PROGRAM P_Prog4
VAR

	fbKL6401 					: FB_LON_KL6401;

	fbREAD_094		: FB_READ_094_SNVT_preset;
	fbSEND_094		: FB_SEND_094_SNVT_preset;

	fbREAD_095		: FB_READ_095_SNVT_switch;
	fbSEND_095		: FB_SEND_095_SNVT_switch;

	fbREAD_096		: FB_READ_096_SNVT_trans_table;
	fbSEND_096		: FB_SEND_096_SNVT_trans_table;

	fbREAD_097		: FB_READ_097_SNVT_override;
	fbSEND_097		: FB_SEND_097_SNVT_override;

	fbREAD_098		: FB_READ_098_SNVT_pwr_fact;
	fbSEND_098		: FB_SEND_098_SNVT_pwr_fact;

	fbREAD_099		: FB_READ_099_SNVT_pwr_fact_f;
	fbSEND_099		: FB_SEND_099_SNVT_pwr_fact_f;

	fbREAD_100		: FB_READ_100_SNVT_density;
	fbSEND_100		: FB_SEND_100_SNVT_density;

	fbREAD_101		: FB_READ_101_SNVT_density_f;
	fbSEND_101		: FB_SEND_101_SNVT_density_f;

	fbREAD_102		: FB_READ_102_SNVT_rpm;
	fbSEND_102		: FB_SEND_102_SNVT_rpm;

	fbREAD_103		: FB_READ_103_SNVT_hvac_emerg;
	fbSEND_103		: FB_SEND_103_SNVT_hvac_emerg;

	fbREAD_104		: FB_READ_104_SNVT_angle_deg;
	fbSEND_104		: FB_SEND_104_SNVT_angle_deg;

	fbREAD_105		: FB_READ_105_SNVT_temp_p;
	fbSEND_105		: FB_SEND_105_SNVT_temp_p;

	fbREAD_106		: FB_READ_106_SNVT_temp_setpt;
	fbSEND_106		: FB_SEND_106_SNVT_temp_setpt;

	fbREAD_107		: FB_READ_107_SNVT_time_sec;
	fbSEND_107		: FB_SEND_107_SNVT_time_sec;

	fbREAD_108		: FB_READ_108_SNVT_hvac_mode;
	fbSEND_108		: FB_SEND_108_SNVT_hvac_mode;

	fbREAD_109		: FB_READ_109_SNVT_occupancy;
	fbSEND_109		: FB_SEND_109_SNVT_occupancy;

	fbREAD_110		: FB_READ_110_SNVT_area;
	fbSEND_110		: FB_SEND_110_SNVT_area;

	fbREAD_111		: FB_READ_111_SNVT_hvac_overid;
	fbSEND_111		: FB_SEND_111_SNVT_hvac_overid;

	fbREAD_112		: FB_READ_112_SNVT_hvac_status;
	fbSEND_112		: FB_SEND_112_SNVT_hvac_status;

	fbREAD_113		: FB_READ_113_SNVT_press_p;
	fbSEND_113		: FB_SEND_113_SNVT_press_p;

	fbREAD_114		: FB_READ_114_SNVT_address;
	fbSEND_114		: FB_SEND_114_SNVT_address;

	fbREAD_115		: FB_READ_115_SNVT_scene;
	fbSEND_115		: FB_SEND_115_SNVT_scene;

	fbREAD_116		: FB_READ_116_SNVT_scene_cfg;
	fbSEND_116		: FB_SEND_116_SNVT_scene_cfg;

	fbREAD_117		: FB_READ_117_SNVT_setting;
	fbSEND_117		: FB_SEND_117_SNVT_setting;

	fbREAD_118		: FB_READ_118_SNVT_evap_state;
	fbSEND_118		: FB_SEND_118_SNVT_evap_state;

	fbREAD_119		: FB_READ_119_SNVT_therm_mode;
	fbSEND_119		: FB_SEND_119_SNVT_therm_mode;

	fbREAD_120		: FB_READ_120_SNVT_defr_mode;
	fbSEND_120		: FB_SEND_120_SNVT_defr_mode;

	fbREAD_121		: FB_READ_121_SNVT_defr_term;
	fbSEND_121		: FB_SEND_121_SNVT_defr_term;

	fbREAD_122		: FB_READ_122_SNVT_defr_state;
	fbSEND_122		: FB_SEND_122_SNVT_defr_state;

	fbREAD_123		: FB_READ_123_SNVT_time_min;
	fbSEND_123		: FB_SEND_123_SNVT_time_min;

	fbREAD_124		: FB_READ_124_SNVT_time_hour;
	fbSEND_124		: FB_SEND_124_SNVT_time_hour;

END_VAR

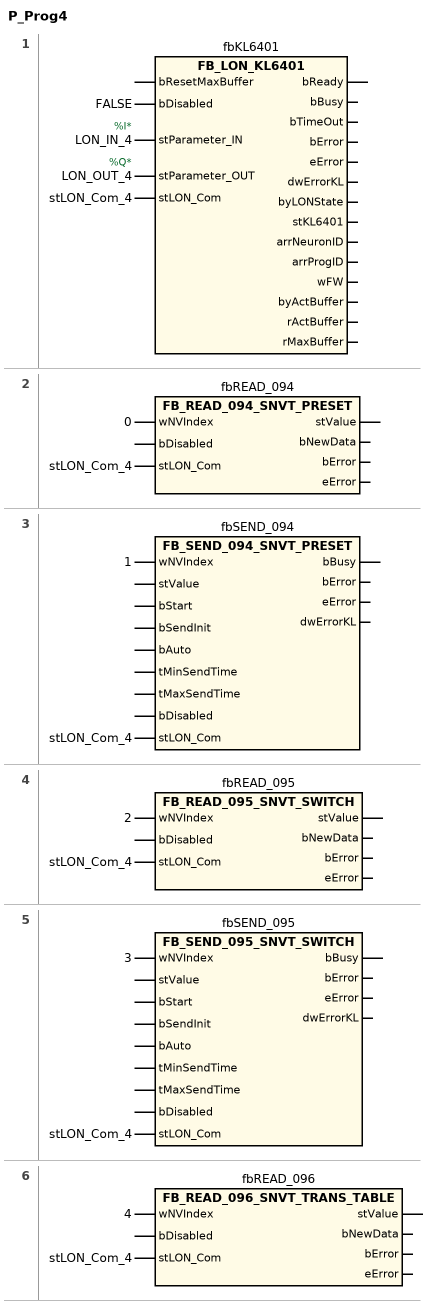
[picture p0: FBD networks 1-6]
// NETWORK 1
//   LON_IN_4: AT %I*
//   LON_OUT_4: AT %Q*
fbKL6401(
    bDisabled := FALSE,
    stParameter_IN := LON_IN_4,
    stParameter_OUT := LON_OUT_4,
    stLON_Com := stLON_Com_4); // FB_LON_KL6401

// NETWORK 2
fbREAD_094(wNVIndex := 0, stLON_Com := stLON_Com_4); // FB_READ_094_SNVT_PRESET

// NETWORK 3
fbSEND_094(wNVIndex := 1, stLON_Com := stLON_Com_4); // FB_SEND_094_SNVT_PRESET

// NETWORK 4
fbREAD_095(wNVIndex := 2, stLON_Com := stLON_Com_4); // FB_READ_095_SNVT_SWITCH

// NETWORK 5
fbSEND_095(wNVIndex := 3, stLON_Com := stLON_Com_4); // FB_SEND_095_SNVT_SWITCH

// NETWORK 6
fbREAD_096(wNVIndex := 4, stLON_Com := stLON_Com_4); // FB_READ_096_SNVT_TRANS_TABLE

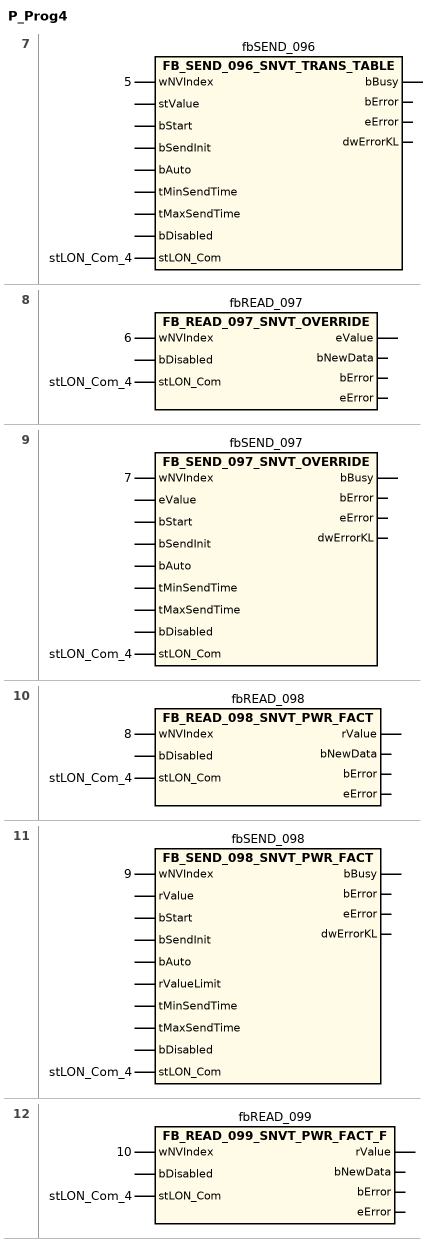
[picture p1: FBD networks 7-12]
// NETWORK 7
fbSEND_096(wNVIndex := 5, stLON_Com := stLON_Com_4); // FB_SEND_096_SNVT_TRANS_TABLE

// NETWORK 8
fbREAD_097(wNVIndex := 6, stLON_Com := stLON_Com_4); // FB_READ_097_SNVT_OVERRIDE

// NETWORK 9
fbSEND_097(wNVIndex := 7, stLON_Com := stLON_Com_4); // FB_SEND_097_SNVT_OVERRIDE

// NETWORK 10
fbREAD_098(wNVIndex := 8, stLON_Com := stLON_Com_4); // FB_READ_098_SNVT_PWR_FACT

// NETWORK 11
fbSEND_098(wNVIndex := 9, stLON_Com := stLON_Com_4); // FB_SEND_098_SNVT_PWR_FACT

// NETWORK 12
fbREAD_099(wNVIndex := 10, stLON_Com := stLON_Com_4); // FB_READ_099_SNVT_PWR_FACT_F

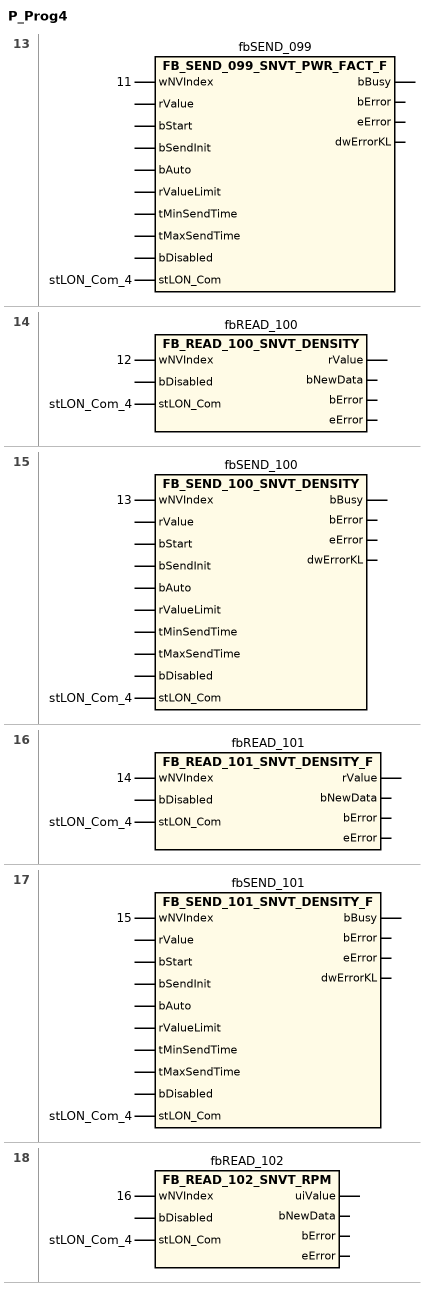
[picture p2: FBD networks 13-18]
// NETWORK 13
fbSEND_099(wNVIndex := 11, stLON_Com := stLON_Com_4); // FB_SEND_099_SNVT_PWR_FACT_F

// NETWORK 14
fbREAD_100(wNVIndex := 12, stLON_Com := stLON_Com_4); // FB_READ_100_SNVT_DENSITY

// NETWORK 15
fbSEND_100(wNVIndex := 13, stLON_Com := stLON_Com_4); // FB_SEND_100_SNVT_DENSITY

// NETWORK 16
fbREAD_101(wNVIndex := 14, stLON_Com := stLON_Com_4); // FB_READ_101_SNVT_DENSITY_F

// NETWORK 17
fbSEND_101(wNVIndex := 15, stLON_Com := stLON_Com_4); // FB_SEND_101_SNVT_DENSITY_F

// NETWORK 18
fbREAD_102(wNVIndex := 16, stLON_Com := stLON_Com_4); // FB_READ_102_SNVT_RPM

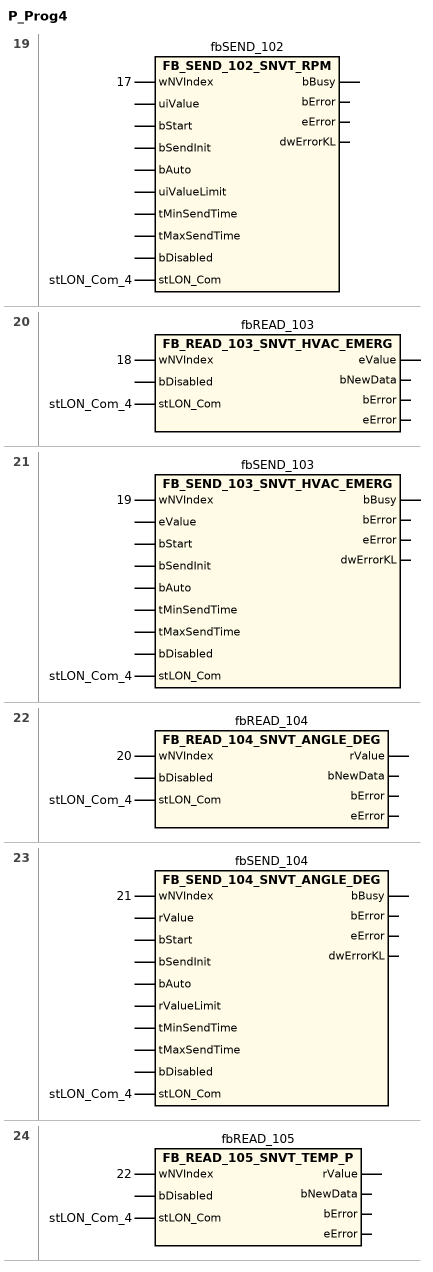
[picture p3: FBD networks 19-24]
// NETWORK 19
fbSEND_102(wNVIndex := 17, stLON_Com := stLON_Com_4); // FB_SEND_102_SNVT_RPM

// NETWORK 20
fbREAD_103(wNVIndex := 18, stLON_Com := stLON_Com_4); // FB_READ_103_SNVT_HVAC_EMERG

// NETWORK 21
fbSEND_103(wNVIndex := 19, stLON_Com := stLON_Com_4); // FB_SEND_103_SNVT_HVAC_EMERG

// NETWORK 22
fbREAD_104(wNVIndex := 20, stLON_Com := stLON_Com_4); // FB_READ_104_SNVT_ANGLE_DEG

// NETWORK 23
fbSEND_104(wNVIndex := 21, stLON_Com := stLON_Com_4); // FB_SEND_104_SNVT_ANGLE_DEG

// NETWORK 24
fbREAD_105(wNVIndex := 22, stLON_Com := stLON_Com_4); // FB_READ_105_SNVT_TEMP_P

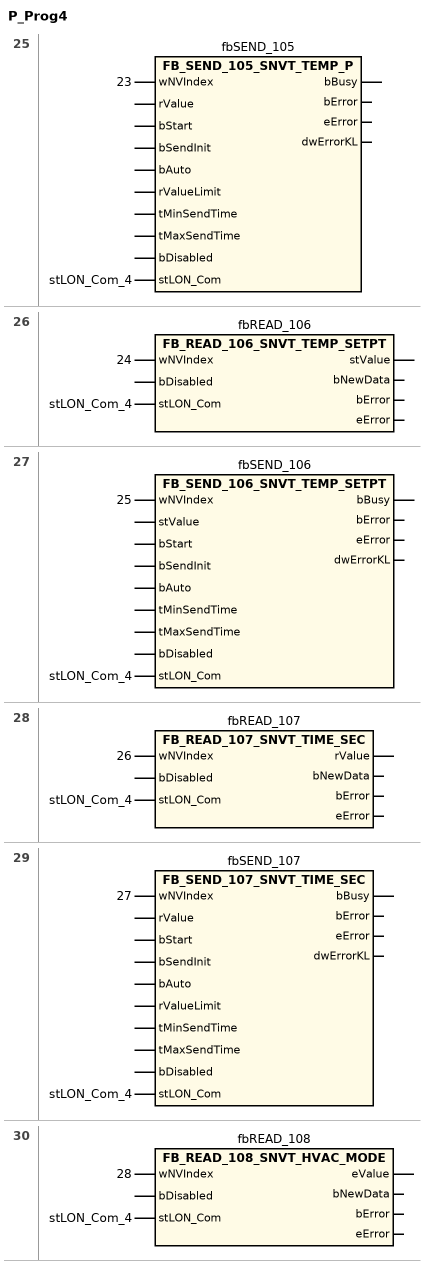
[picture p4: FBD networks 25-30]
// NETWORK 25
fbSEND_105(wNVIndex := 23, stLON_Com := stLON_Com_4); // FB_SEND_105_SNVT_TEMP_P

// NETWORK 26
fbREAD_106(wNVIndex := 24, stLON_Com := stLON_Com_4); // FB_READ_106_SNVT_TEMP_SETPT

// NETWORK 27
fbSEND_106(wNVIndex := 25, stLON_Com := stLON_Com_4); // FB_SEND_106_SNVT_TEMP_SETPT

// NETWORK 28
fbREAD_107(wNVIndex := 26, stLON_Com := stLON_Com_4); // FB_READ_107_SNVT_TIME_SEC

// NETWORK 29
fbSEND_107(wNVIndex := 27, stLON_Com := stLON_Com_4); // FB_SEND_107_SNVT_TIME_SEC

// NETWORK 30
fbREAD_108(wNVIndex := 28, stLON_Com := stLON_Com_4); // FB_READ_108_SNVT_HVAC_MODE

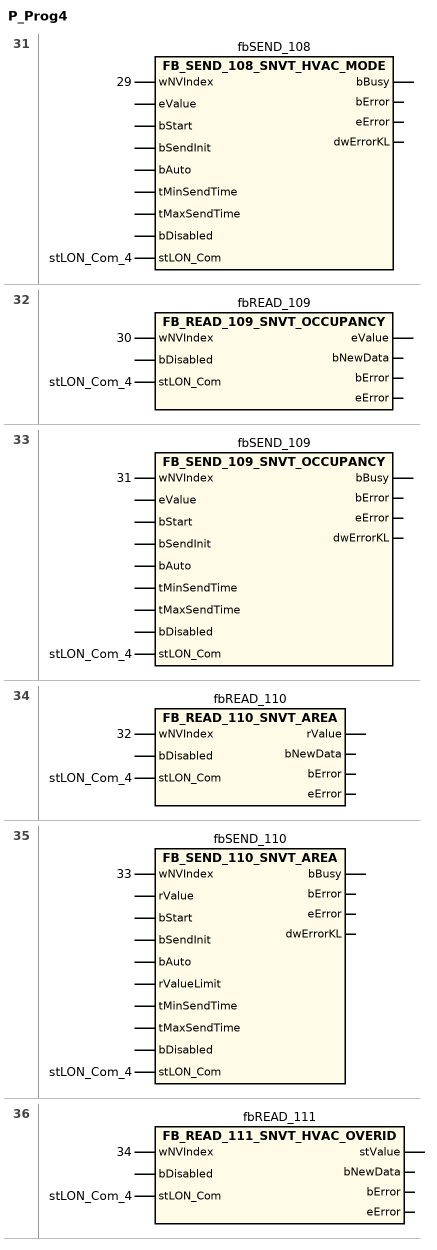
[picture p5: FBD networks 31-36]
// NETWORK 31
fbSEND_108(wNVIndex := 29, stLON_Com := stLON_Com_4); // FB_SEND_108_SNVT_HVAC_MODE

// NETWORK 32
fbREAD_109(wNVIndex := 30, stLON_Com := stLON_Com_4); // FB_READ_109_SNVT_OCCUPANCY

// NETWORK 33
fbSEND_109(wNVIndex := 31, stLON_Com := stLON_Com_4); // FB_SEND_109_SNVT_OCCUPANCY

// NETWORK 34
fbREAD_110(wNVIndex := 32, stLON_Com := stLON_Com_4); // FB_READ_110_SNVT_AREA

// NETWORK 35
fbSEND_110(wNVIndex := 33, stLON_Com := stLON_Com_4); // FB_SEND_110_SNVT_AREA

// NETWORK 36
fbREAD_111(wNVIndex := 34, stLON_Com := stLON_Com_4); // FB_READ_111_SNVT_HVAC_OVERID

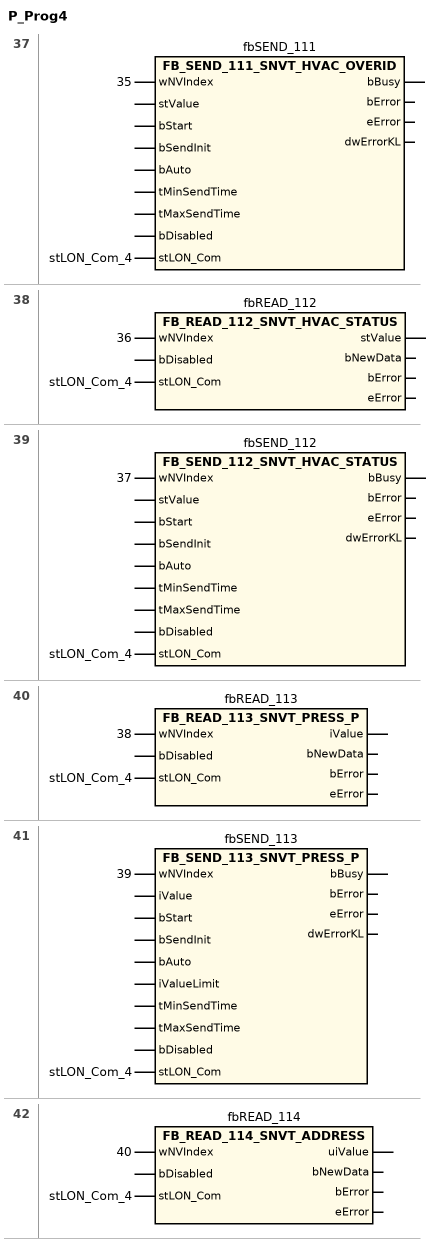
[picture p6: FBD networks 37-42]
// NETWORK 37
fbSEND_111(wNVIndex := 35, stLON_Com := stLON_Com_4); // FB_SEND_111_SNVT_HVAC_OVERID

// NETWORK 38
fbREAD_112(wNVIndex := 36, stLON_Com := stLON_Com_4); // FB_READ_112_SNVT_HVAC_STATUS

// NETWORK 39
fbSEND_112(wNVIndex := 37, stLON_Com := stLON_Com_4); // FB_SEND_112_SNVT_HVAC_STATUS

// NETWORK 40
fbREAD_113(wNVIndex := 38, stLON_Com := stLON_Com_4); // FB_READ_113_SNVT_PRESS_P

// NETWORK 41
fbSEND_113(wNVIndex := 39, stLON_Com := stLON_Com_4); // FB_SEND_113_SNVT_PRESS_P

// NETWORK 42
fbREAD_114(wNVIndex := 40, stLON_Com := stLON_Com_4); // FB_READ_114_SNVT_ADDRESS

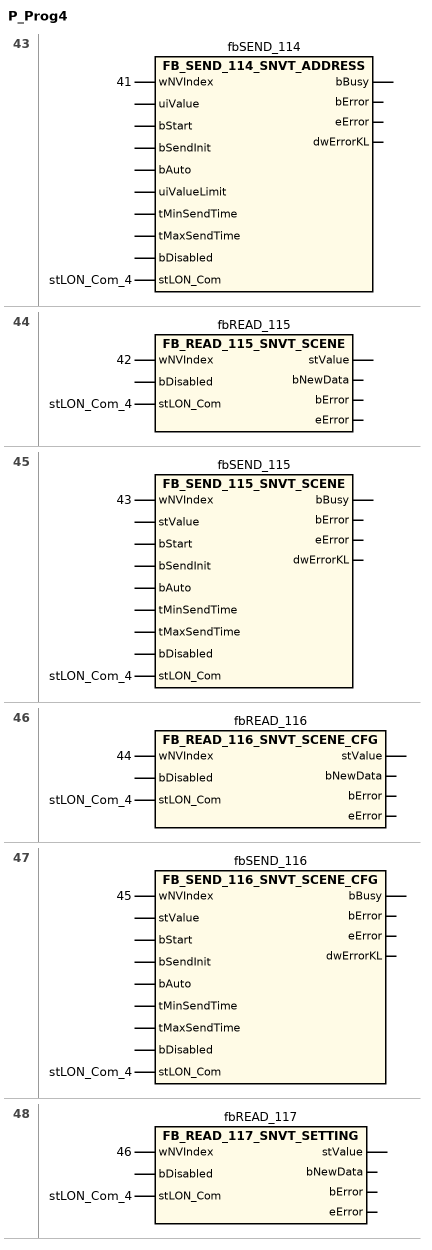
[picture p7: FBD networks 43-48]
// NETWORK 43
fbSEND_114(wNVIndex := 41, stLON_Com := stLON_Com_4); // FB_SEND_114_SNVT_ADDRESS

// NETWORK 44
fbREAD_115(wNVIndex := 42, stLON_Com := stLON_Com_4); // FB_READ_115_SNVT_SCENE

// NETWORK 45
fbSEND_115(wNVIndex := 43, stLON_Com := stLON_Com_4); // FB_SEND_115_SNVT_SCENE

// NETWORK 46
fbREAD_116(wNVIndex := 44, stLON_Com := stLON_Com_4); // FB_READ_116_SNVT_SCENE_CFG

// NETWORK 47
fbSEND_116(wNVIndex := 45, stLON_Com := stLON_Com_4); // FB_SEND_116_SNVT_SCENE_CFG

// NETWORK 48
fbREAD_117(wNVIndex := 46, stLON_Com := stLON_Com_4); // FB_READ_117_SNVT_SETTING

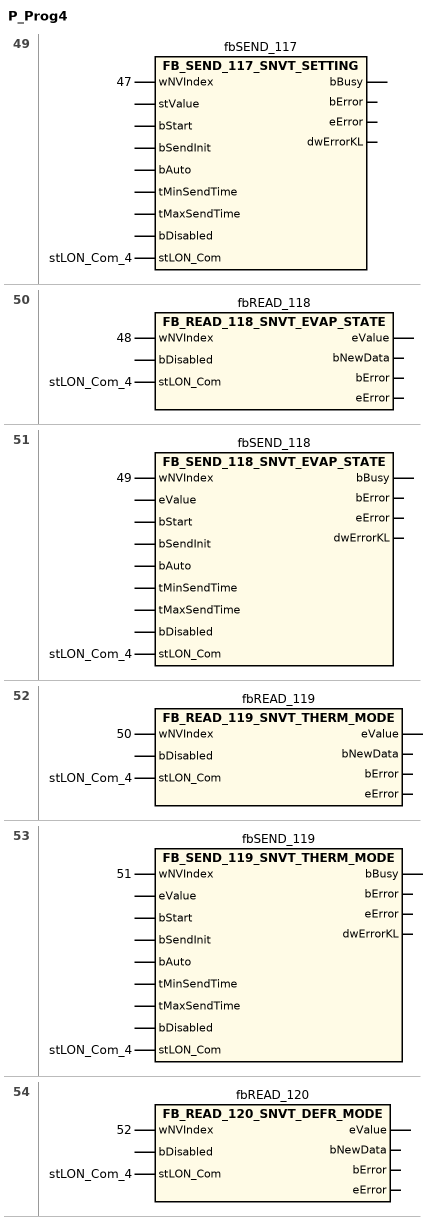
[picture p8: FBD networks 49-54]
// NETWORK 49
fbSEND_117(wNVIndex := 47, stLON_Com := stLON_Com_4); // FB_SEND_117_SNVT_SETTING

// NETWORK 50
fbREAD_118(wNVIndex := 48, stLON_Com := stLON_Com_4); // FB_READ_118_SNVT_EVAP_STATE

// NETWORK 51
fbSEND_118(wNVIndex := 49, stLON_Com := stLON_Com_4); // FB_SEND_118_SNVT_EVAP_STATE

// NETWORK 52
fbREAD_119(wNVIndex := 50, stLON_Com := stLON_Com_4); // FB_READ_119_SNVT_THERM_MODE

// NETWORK 53
fbSEND_119(wNVIndex := 51, stLON_Com := stLON_Com_4); // FB_SEND_119_SNVT_THERM_MODE

// NETWORK 54
fbREAD_120(wNVIndex := 52, stLON_Com := stLON_Com_4); // FB_READ_120_SNVT_DEFR_MODE

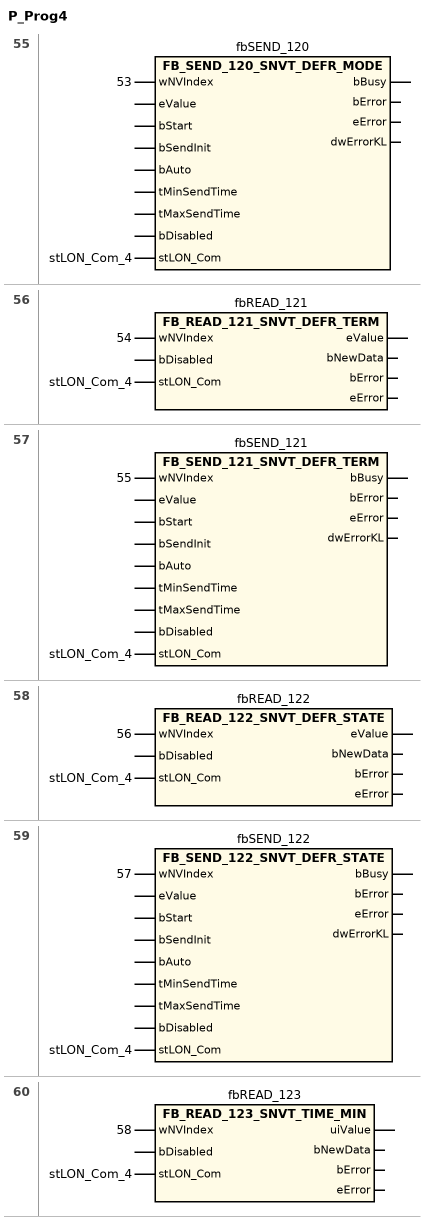
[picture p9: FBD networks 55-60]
// NETWORK 55
fbSEND_120(wNVIndex := 53, stLON_Com := stLON_Com_4); // FB_SEND_120_SNVT_DEFR_MODE

// NETWORK 56
fbREAD_121(wNVIndex := 54, stLON_Com := stLON_Com_4); // FB_READ_121_SNVT_DEFR_TERM

// NETWORK 57
fbSEND_121(wNVIndex := 55, stLON_Com := stLON_Com_4); // FB_SEND_121_SNVT_DEFR_TERM

// NETWORK 58
fbREAD_122(wNVIndex := 56, stLON_Com := stLON_Com_4); // FB_READ_122_SNVT_DEFR_STATE

// NETWORK 59
fbSEND_122(wNVIndex := 57, stLON_Com := stLON_Com_4); // FB_SEND_122_SNVT_DEFR_STATE

// NETWORK 60
fbREAD_123(wNVIndex := 58, stLON_Com := stLON_Com_4); // FB_READ_123_SNVT_TIME_MIN

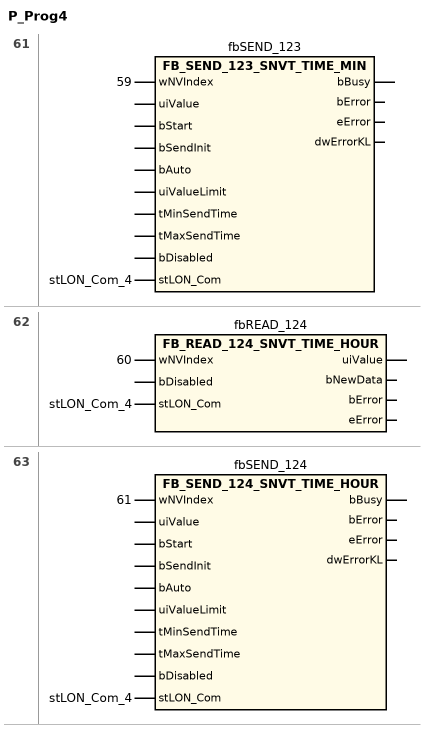
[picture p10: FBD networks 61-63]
// NETWORK 61
fbSEND_123(wNVIndex := 59, stLON_Com := stLON_Com_4); // FB_SEND_123_SNVT_TIME_MIN

// NETWORK 62
fbREAD_124(wNVIndex := 60, stLON_Com := stLON_Com_4); // FB_READ_124_SNVT_TIME_HOUR

// NETWORK 63
fbSEND_124(wNVIndex := 61, stLON_Com := stLON_Com_4); // FB_SEND_124_SNVT_TIME_HOUR

END_PROGRAM
